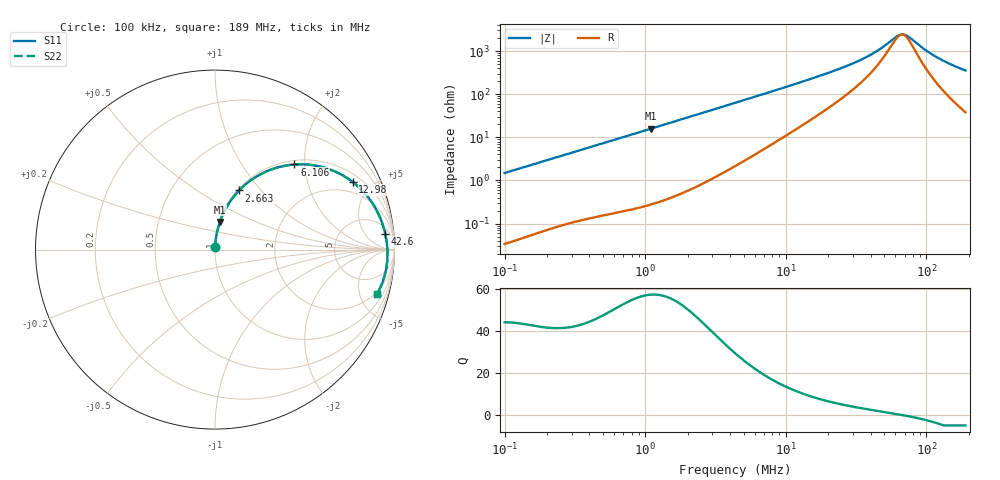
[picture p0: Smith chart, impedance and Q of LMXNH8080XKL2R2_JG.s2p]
! LMXNH8080XKL2R2_JG  S-PARAMETER MODEL  ( General Type )
! Model Generated by TAIYO YUDEN Corporation (https://www.yuden.co.jp/en/)
! Version 1.0
! TAIYO YUDEN Control No. 191025NI43SB-FBB
! Copyright(c) 2019 TAIYO YUDEN CO.,LTD. All Rights Reserved.
! Product Description (link to TY-COMPAS)
! https://ds.yuden.co.jp/TYCOMPAS/or/detail?pn=LMXNH8080XKL2R2NJG&u=M
! Products Name : Inductors
! Characteristics :
!  Inductance : 2.2 uH , SRF(min) : 60 MHz , DC Resistance(max) : 0.0195 Ohm
!  Rated Current : Saturation :4900 mA , Temp Rise : 4800 mA (40 degC)
!  Case Size : 8.0 x 8.0 / 0.315 x 0.315 [mm/inch] , Thickness : 3 / 0.118 [mm/inch]
!  (Conditions: Temperature = 25 degC , DC Bias Current/Voltage = 0A / 0V)
! External Node Assignments :
!  1  o---GGG---o  2
! GND o---------o GND
! Frequency Range : 0.1MHz  -  189.042664MHz  [ 402 STEP ]
# MHz S RI R 50
! Freq[MHz].  S11 Real  S11 Imag  S21 Real  S21 Imag  S12 Real  S12 Imag  S22 Real  S22 Imag
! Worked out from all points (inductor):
!   401 points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, 100 kHz to 189 MHz, reference 50 ohm
!   read as one part in series: L = 2.36 uH near 103.8 kHz
!   highest Q = 57.2 at 1.097 MHz (marker M1), where L = 2.3 uH
!   self-resonance near 66.78 MHz
!   S11 on the Smith chart (normalised r, x): 100 kHz: 1.00, +0.03; 2.663 MHz: 1.02, +0.77; 6.106 MHz: 1.08, +1.77; 12.98 MHz: 1.37, +3.84; 42.6 MHz: 9, +17; 189 MHz: 1.76, -7.04
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0.1  0.000559 0.0149  0.9994 -0.0149  0.9994 -0.0149  0.000559 0.0149
0.353854  0.00386 0.0514  0.9961 -0.0514  0.9961 -0.0514  0.00386 0.0514
1.097255  0.0271 0.1538  0.9729 -0.1538  0.9729 -0.1538  0.0271 0.1538
1.252125  0.0345 0.174  0.9655 -0.174  0.9655 -0.174  0.0345 0.174
1.896087  0.0739 0.2521  0.9261 -0.2521  0.9261 -0.2521  0.0739 0.2521
2.662585  0.1345 0.3297  0.8655 -0.3297  0.8655 -0.3297  0.1345 0.3297
4.347904  0.2899 0.437  0.7101 -0.437  0.7101 -0.437  0.2899 0.437
6.105554  0.4425 0.4741  0.5575 -0.4741  0.5575 -0.4741  0.4425 0.4741
8.57374  0.6043 0.4581  0.3957 -0.4581  0.3957 -0.4581  0.6043 0.4581
12.98318  0.7675 0.3767  0.2325 -0.3767  0.2325 -0.3767  0.7675 0.3767
15.38522  0.8166 0.3333  0.1834 -0.3333  0.1834 -0.3333  0.8166 0.3333
27.60814  0.9172 0.1842  0.0828 -0.1842  0.0828 -0.1842  0.9172 0.1842
42.60291  0.948 0.0894  0.052 -0.0894  0.052 -0.0894  0.948 0.0894
54.44117  0.9567 0.0404  0.0433 -0.0404  0.0433 -0.0404  0.9567 0.0404
63.30801  0.9597 0.0106  0.0403 -0.0106  0.0403 -0.0106  0.9597 0.0106
66.99353  0.9604 -0.000647  0.0396 0.000647  0.0396 0.000647  0.9604 -0.000647
70.8936  0.9608 -0.012  0.0392 0.012  0.0392 0.012  0.9608 -0.012
76.44915  0.961 -0.0273  0.039 0.0273  0.039 0.0273  0.961 -0.0273
97.69241  0.9579 -0.0794  0.0421 0.0794  0.0421 0.0794  0.9579 -0.0794
115.7666  0.9516 -0.1183  0.0484 0.1183  0.0484 0.1183  0.9516 -0.1183
147.9352  0.9341 -0.1795  0.0659 0.1795  0.0659 0.1795  0.9341 -0.1795
189.0427  0.9033 -0.2463  0.0967 0.2463  0.0967 0.2463  0.9033 -0.2463
